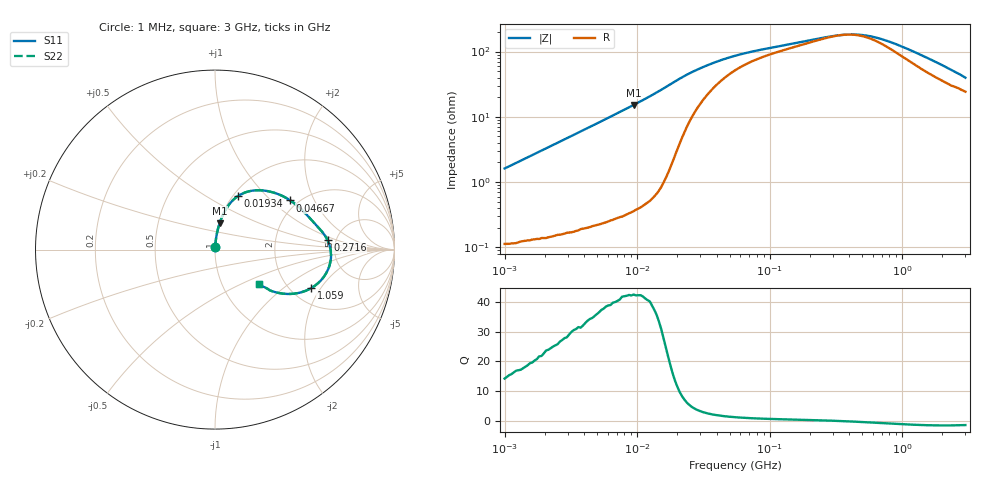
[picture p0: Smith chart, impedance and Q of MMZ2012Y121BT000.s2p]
! S-parameter Generated by TDK Corporation
! Copyright(C) 2016 TDK Corporation.
! All Rights Reserved.
! TDK P/N: MMZ2012Y121BT000 (Chip Beads)
! Property: |Z|=120¶ at 100MHz
! Size(LxWxT): 2x1.25x0.85mm, 0.079x0.049x0.033inches
! Model Type: s2p (Touchstone File Format Version 1.0)
! Frequency: DC=Yes Start=1MHz Stop=3000MHz 202points Log-sweep
! Note: This model was converted from impedance.
! Model Generated on May. 16, 2016
! Hash(MD5):
! Port Assignments:
!  1 ---@@@--- 2
! Applicable Conditions:
!  Temperature = 25 degC
!  DC Bias Current = 0 A
!  Small Signal Operation
! Terms and conditions regarding TDK Simulation Models
! (1)This simulation model is being provided solely for informational purposes. Please refer to the specifications of the products in terms of detailed characteristics of such products.
! (2)In no event shall TDK Corporation of any of its subsidiaries be liable for any loss or damage arising, directly or indirectly,
!  From any information contained in this simulation model, including, but not limited to loss or damages arising from any inaccuracies, omissions or errors in connection with such information.
! (3)Any and all copyrights on this simulation model are owned by TDK Corporation.
!  Duplication or redistribution of this simulation model without prior written permission from TDK Corporation is prohibited.
! (4)This simulation model is subject to any modification or change without any prior notice.
! (5)Neither TDK Corporation nor any of its subsidiaries shall make any warranty, express or implied,
!  Including but not limited to the correctness, implied warranties of merchantability and fitness for a particular purpose with respect to this simulation models.
! (6)The use of this simulation model shall be deemed to have consented to the terms and conditions hereof.
# MHz S MA R 50
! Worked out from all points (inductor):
!   201 points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, 1 MHz to 3 GHz, reference 50 ohm
!   read as one part in series: L = 256 nH near 1.041 MHz
!   highest Q = 42.2 at 9.41 MHz (marker M1), where L = 257 nH
!   self-resonance near 369.6 MHz
!   S11 on the Smith chart (normalised r, x): 1 MHz: 1.00, +0.03; 19.34 MHz: 1.05, +0.70; 46.67 MHz: 1.82, +1.33; 271.6 MHz: 4.25, +0.75; 1.059 GHz: 2.55, -1.64; 3 GHz: 1.49, -0.63
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1  0.01614 85.1  0.9987 -0.9  0.9987 -0.9  0.01614 85.1
3.900413  0.06182 84.7  0.9962 -3.5  0.9962 -3.5  0.06182 84.7
9.410094  0.1497 80.0  0.9852 -8.6  0.9852 -8.6  0.1497 80.0
14.61624  0.2384 74.5  0.964 -13.8  0.964 -13.8  0.2384 74.5
19.34349  0.322 67.0  0.9232 -18.7  0.9232 -18.7  0.322 67.0
22.70269  0.3704 60.6  0.8797 -21.5  0.8797 -21.5  0.3704 60.6
27.73354  0.4193 52.0  0.8118 -24.0  0.8118 -24.0  0.4193 52.0
36.70325  0.4698 41.0  0.7151 -25.5  0.7151 -25.5  0.4698 41.0
46.66789  0.501 33.1  0.6419 -25.3  0.6419 -25.3  0.501 33.1
54.77226  0.517 28.8  0.6009 -24.5  0.6009 -24.5  0.517 28.8
88.54986  0.5526 19.3  0.5121 -20.9  0.5121 -20.9  0.5526 19.3
213.6344  0.6129 8.1  0.4026 -12.4  0.4026 -12.4  0.6129 8.1
271.6345  0.6291 4.9  0.3769 -8.1  0.3769 -8.1  0.6291 4.9
374.1707  0.6446 -0.2  0.3555 0.4  0.3555 0.4  0.6446 -0.2
475.755  0.6476 -4.6  0.3582 8.3  0.3582 8.3  0.6476 -4.6
604.9187  0.6408 -9.4  0.3823 15.9  0.3823 15.9  0.6408 -9.4
800.5644  0.6182 -15.5  0.4365 22.2  0.4365 22.2  0.6182 -15.5
1059.487  0.5776 -21.8  0.5107 24.8  0.5107 24.8  0.5776 -21.8
1402.151  0.5196 -27.9  0.5926 24.2  0.5926 24.2  0.5196 -27.9
1782.824  0.4592 -32.4  0.6601 21.9  0.6601 21.9  0.4592 -32.4
2266.846  0.3917 -36.2  0.7218 18.7  0.7218 18.7  0.3917 -36.2
3000  0.3098 -38.1  0.7802 14.2  0.7802 14.2  0.3098 -38.1
